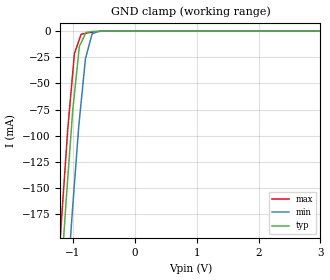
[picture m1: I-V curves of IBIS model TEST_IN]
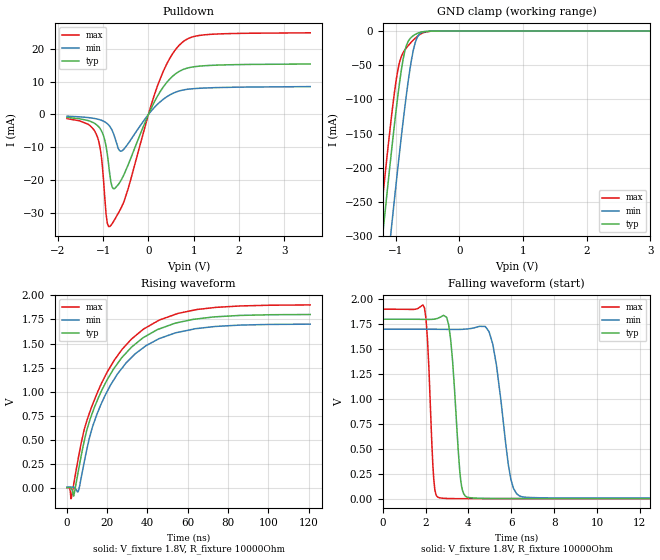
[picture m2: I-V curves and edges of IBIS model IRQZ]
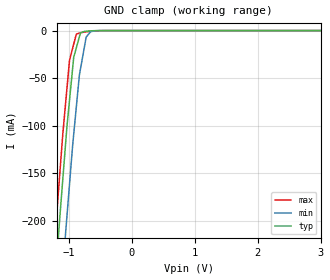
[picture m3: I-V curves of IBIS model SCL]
|Texas Instruments Incorporated
|Ultra low power, High performance DirectPath Class-G headphone amplifier
| part#   Voltage Range(Digital)   Package-type   #pin
|TPA6166A2   1.7V to 1.9V   25-ball WCSP   25
[IBIS Ver]   4.1
[File name]   tpa6166a2.ibs
[File Rev]   1.0
[Date]   02/25/2014
[Source]   Texas Instruments Incorporated.
   Analog-eLab, HPA
   12500 TI Blvd
   Dallas, TX -75243
   For Support e-mail: elab_ibis@list.ti.com
[Notes]   Revision History:
   1.0: 02/25/2014
   - Initial version of the model
   - Initial Model generated from simulations.
   - Model not matched to measurements
   - ccomp values are based on PVT conditions although listed
   in numerical order
   - Pull dowon non-monotinicity in SDA and IRQZ reflects
   the behavior based on simulations
[Disclaimer]
 This product is designed as an aid for customers of Texas Instruments.
 No warranties, either expressed or implied, with respect to this third
 party software (if any) or with respect to its fitness for any
 particular purpose is claimed by Texas Instruments or the author. The
 software (if any) is provided solely on an "as is" basis. The entire
 risk as to its quality and performance is with the customer
[Copyright] (C) Copyright 2014 Texas Instruments Incorporated.
   All rights reserved.
|   TPA6166A2
[Component]   tpa6166a2
[Manufacturer] TI
[Package]   | 20 pin  package
| variable   typ   min   max
R_pkg   0.01   NA   NA
L_pkg   0.1nH   NA   NA
C_pkg   0.1pF   NA   NA
|-------------------------PIN------------------------------------------------
[Pin] signal_name  model_name  R_pin  L_pin C_pin
A1   GND1   GND   NA   NA   NA
A2   INR   TERM   NA   NA   NA
A3   INL   TERM   NA   NA   NA
A4   CPVDD   POWER   NA   NA   NA
A5   JACK_SENSE   TERM   NA   NA   NA
B1   NC   NC   NA   NA   NA
B2   GND2   TERM   NA   NA   NA
B3   IRQB   IRQZ   NA   NA   NA
B4   MOUTN   TERM   NA   NA   NA
B5   TIP   TERM   NA   NA   NA
C1   CPVSS   GND   NA   NA   NA
C2   SCL   SCL   NA   NA   NA
C3   GND   GND   NA   NA   NA
C4   MOUTP   TERM   NA   NA   NA
C5   RING1   TERM   NA   NA   NA
D1   C1N   TERM   NA   NA   NA
D2   SDA   SDA   NA   NA   NA
D3   PGND   GND   NA   NA   NA
D4   NC   NC   NA   NA   NA
D5   MICVDD   POWER   NA   NA   NA
E1   C1P   TERM   NA   NA   NA
E2   PGND   GND   NA   NA   NA
E3   VDD   POWER   NA   NA   NA
E4   RING2   TERM   NA   NA   NA
E5   SLEEVE   TERM   NA   NA   NA
|   TERM Model
[Model] TERM
Model_type Terminator
C_comp   0   0   0
| variable   typ   min   max
[Voltage Range]   3.0V   2.4V   3.6V
[POWER Clamp Reference]  3.0V   2.4V   3.6V
[GND Clamp Reference]   0.0V   0.0V   0.0V
|Operating Temperature
[Temperature Range]   27   125   -25
| Models and submodels in the file (5): TEST_IN (Input), IRQZ (I/O_open_drain), SCL (Input), SDA (I/O_open_drain), TERM (Terminator)
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|   EXT_CLK
[Model]   TEST_IN
Model_type   Input
Vinl = 0.4
Vinh = 1.4
|   typ   min   max
C_comp   0.84818527pF  0.843495394pF  0.860082522pF
[Voltage Range]   1.8   1.7   1.9
[Temperature Range]   27   125   -25
[Power Clamp Reference]   1.8   1.7   1.9
[GND Clamp Reference]   -0   -0   -0
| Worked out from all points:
|   GND clamp passes 1 mA (typ) near -0.75 V on its own axis
[GND Clamp]
|   Voltage   I(typ)   I(min)   I(max)
-1.8V     -811.2mA   -906.5mA   -765.4mA
-1.19V    -234.8mA   -332.3mA   -186.8mA
-1.12V    -172.7mA   -269.2mA   -126.7mA
-1.082V   -141.2mA   -236.5mA   -94.17mA
-1.012V   -84.35mA   -176mA     -47.05mA
-974.4mV  -60.31mA   -146.2mA   -21.55mA
-894.6mV  -14.6mA    -85.29mA   -7.914mA
-866.4mV  -11.13mA   -68.41mA   -3.089mA
-796.3mV  -2.514mA   -26.5mA    -2.137mA
-688.3mV  -441.3uA   -2.539mA   -1.018mA
-580.3mV  -91.85uA   -161.8uA   -340.5uA
3.6V      0A         0A         0A
[POWER Clamp]
|   Voltage   I(typ)   I(min)   I(max)
-1.8V     0A         0A         0A
0V        0A         0A         0A
3.6V      0A         0A         0A
|   IRQZ
[Model]   IRQZ
Model_type   I/O_open_drain
Polarity   Non-Inverting
Enable   Active-Low
Vinl = 0.4
Vinh = 1.4
Vmeas = 0.9
Vref = 0.9
Cref = 1pF
Rref = 10000
|   typ   min   max
C_comp   1.5307pF  1.303pF   1.7195pF
[Voltage Range]   1.8   1.7   1.9
[Temperature Range]   27   125   -25
[Pullup Reference]   1.8   1.7   1.9
[Pulldown Reference]   -0   -0   -0
[Power Clamp Reference]   1.8   1.7   1.9
[GND Clamp Reference]   -0   -0   -0
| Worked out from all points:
|   slope of the pulldown table from 0 to 0.27 V, typ, clamps not added: 37.5 ohm
|   GND clamp passes 1 mA (typ) near -0.57 V on its own axis
|   falling waveform, V_fixture 1.8V, R_fixture 10000Ohm: 20-80 % time 331ps typ, 570ps min, 224ps max; typ from 1.8 V to 0.006 V
|   rising waveform, V_fixture 1.8V, R_fixture 10000Ohm: 20-80 % time 23.8ns typ, 23.1ns min, 24.7ns max; typ from 0.006 V to 1.8 V
[Pulldown]
|   Voltage   I(typ)   I(min)   I(max)
-1.8V     -909.1uA   -538uA     -1.278mA
-1.341V   -1.83mA    -936uA     -2.938mA
-1.125V   -3.387mA   -1.422mA   -6.928mA
-1.044V   -4.84mA    -1.756mA   -12.37mA
-909mV    -12.08mA   -2.811mA   -33.21mA
-855mV    -18.17mA   -3.613mA   -34.26mA
-774mV    -22.7mA    -5.767mA   -32.75mA
-585mV    -19.6mA    -11.14mA   -28.02mA
198mV     5.552mA    3.077mA    8.653mA
684mV     13.18mA    7.198mA    21.2mA
1.224V    14.87mA    8.064mA    24.3mA
3.573V    15.41mA    8.504mA    24.94mA
[GND Clamp]
|   Voltage   I(typ)   I(min)   I(max)
-1.8V     -867.5mA   -980.2mA   -812.8mA
-1.287V   -377.2mA   -491.3mA   -321.8mA
-1.233V   -327.1mA   -441.1mA   -272mA
-1.179V   -277.7mA   -391.3mA   -223.2mA
-1.071V   -181.8mA   -293.4mA   -130.5mA
-963mV    -93.85mA   -199.1mA   -56.44mA
-882mV    -41.5mA    -132.5mA   -31.71mA
-774mV    -11.18mA   -55.6mA    -18.4mA
-693mV    -5.048mA   -17.45mA   -10.66mA
-612mV    -1.86mA    -3.316mA   -4.741mA
-450mV    -113uA     -165.5uA   -237.9uA
3.573V    0A         0A         0A
[POWER Clamp]
|   Voltage   I(typ)   I(min)   I(max)
-1.8V     0A         0A         0A
0V        0A         0A         0A
3.6V      0A         0A         0A
[Ramp]
R_load = 10000
|   typ   min   max
dV/dt_r   1.07735/2.37803e-008   1.01477/2.30726e-008   1.13808/2.46514e-008
dV/dt_f   1.07662/3.31194e-010   1.01415/5.70145e-010   1.1377/2.24303e-010
[Falling Waveform]
V_fixture = 1.8V
V_fixture_min = 1.7V
V_fixture_max = 1.9V
R_fixture = 10000Ohm
C_fixture = 0F
|   Time   V(typ)   V(min)   V(max)
0s        1.8V       1.7V       1.9V
1.943ns   1.798V     1.7V       1.915V
2.428ns   1.802V     1.7V       96.62mV
2.9ns     1.83V      1.699V     7.172mV
3.675ns   131.3mV    1.699V     4.299mV
4.243ns   10.6mV     1.713V     4.24mV
4.959ns   6.485mV    1.677V     4.203mV
5.979ns   6.035mV    197mV      4.149mV
6.692ns   6.018mV    18.12mV    4.111mV
120.8ns   5.638mV    9.579mV    3.85mV
[Rising Waveform]
V_fixture = 1.8V
V_fixture_min = 1.7V
V_fixture_max = 1.9V
R_fixture = 10000Ohm
C_fixture = 0F
|   Time   V(typ)   V(min)   V(max)
0s        5.635mV    9.572mV    3.875mV
2.083ns   3.056mV    10.05mV    -110.2mV
3.351ns   -81.46mV   8.56mV     37.52mV
5.523ns   162.2mV    -38mV      296.5mV
9.754ns   594.9mV    389.7mV    689.9mV
17.13ns   1.007V     878.9mV    1.086V
25.14ns   1.293V     1.185V     1.375V
38.02ns   1.563V     1.458V     1.65V
64.6ns    1.755V     1.656V     1.853V
120.8ns   1.801V     1.701V     1.901V
|   SCL
[Model]   SCL
Model_type   Input
Vinl = 0.4
Vinh = 1.4
|   typ   min   max
C_comp   0.8513pF  0.8434pF   0.8631pF
[Voltage Range]   1.8   1.7   1.9
[Temperature Range]   27   125   -25
[Power Clamp Reference]   1.8   1.7   1.9
[GND Clamp Reference]   -0   -0   -0
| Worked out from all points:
|   GND clamp passes 1 mA (typ) near -0.76 V on its own axis
[GND Clamp]
|   Voltage   I(typ)   I(min)   I(max)
-1.8V     -811.2mA   -906.5mA   -765.4mA
-1.251V   -289.4mA   -387.3mA   -242.1mA
-1.21V    -252.1mA   -349.7mA   -204.1mA
-1.16V    -208mA     -305mA     -161.2mA
-1.052V   -116mA     -210mA     -74.15mA
-993.6mV  -73.3mA    -161.6mA   -31.3mA
-927mV    -28.2mA    -109.2mA   -14.29mA
-885.6mV  -18.3mA    -80.62mA   -3.713mA
-836.5mV  -6.553mA   -46.72mA   -2.709mA
-728.5mV  -681.4uA   -6.85mA    -1.349mA
-657.3mV  -289.1uA   -1.148mA   -754.1uA
3.6V      0A         0A         0A
[POWER Clamp]
|   Voltage   I(typ)   I(min)   I(max)
-1.8V     0A         0A         0A
0V        0A         0A         0A
3.6V      0A         0A         0A
